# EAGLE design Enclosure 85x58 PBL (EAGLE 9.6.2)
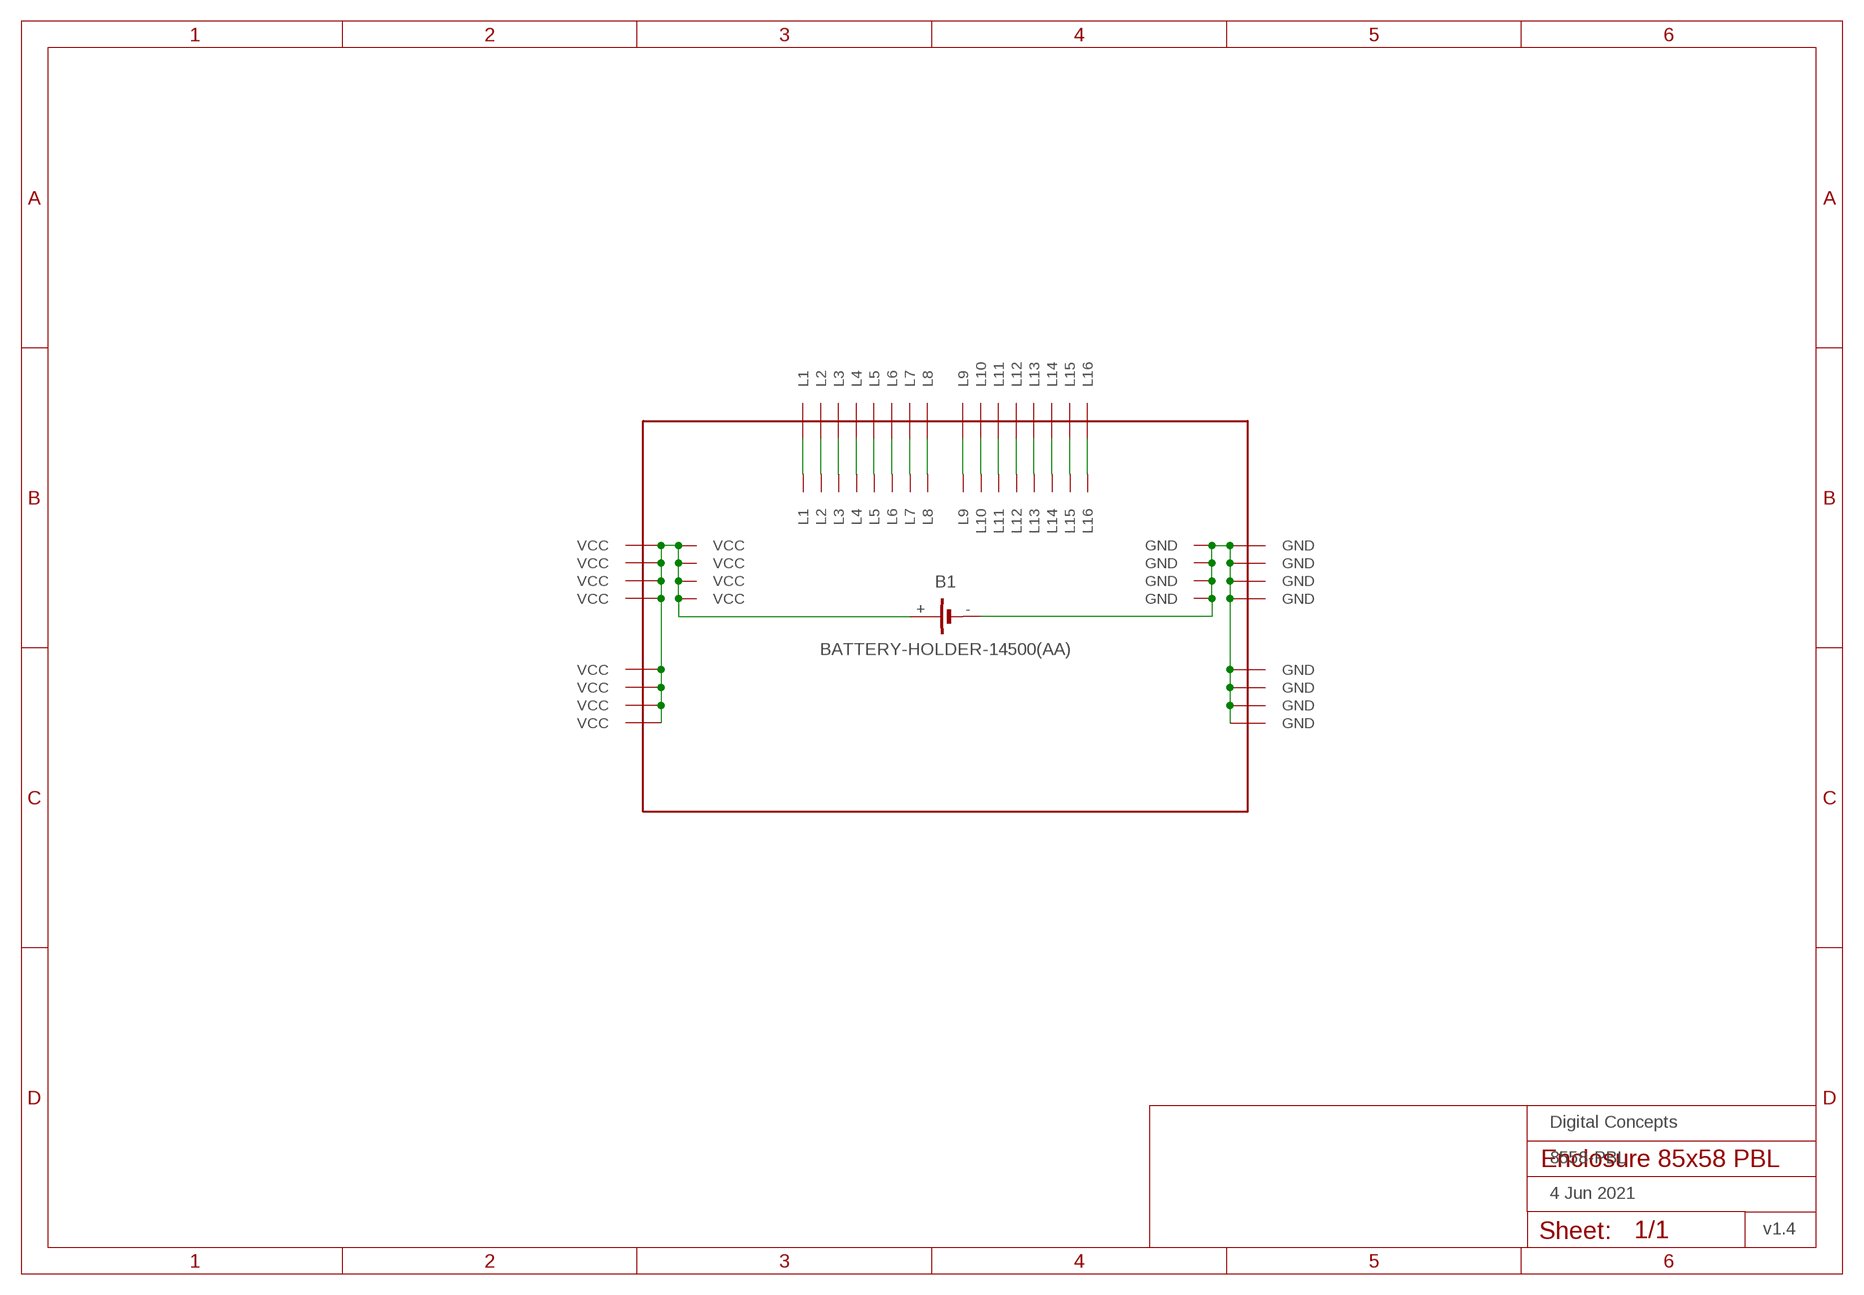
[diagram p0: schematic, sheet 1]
FRAME1 (FRAME-A4L-LOC): DATE: 4 Jun 2021; OWNER: Digital Concepts; TITLE: 8558-PBL; VERSION: v1.4

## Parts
B1  BATTERY-HOLDER-14500(AA)  [BATTERY-14500]
U$1  PROTO-28X18-BAT  [PROTO-28X18-BAT]

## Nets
GND: B1.- U$1.P27-12(GND) U$1.P27-13(GND) U$1.P27-14(GND) U$1.P27-15(GND) U$1.P28-04(GND) U$1.P28-05(GND) U$1.P28-06(GND) U$1.P28-07(GND) U$1.P28-12(GND) U$1.P28-13(GND) U$1.P28-14(GND) U$1.P28-15(GND)
N$4: U$1.P07-17(L1) U$1.P07-18(L1)
N$5: U$1.P08-17(L2) U$1.P08-18(L2)
N$6: U$1.P09-17(L3) U$1.P09-18(L3)
N$7: U$1.P10-17(L4) U$1.P10-18(L4)
N$8: U$1.P11-17(L5) U$1.P11-18(L5)
N$9: U$1.P12-17(L6) U$1.P12-18(L6)
N$10: U$1.P13-17(L7) U$1.P13-18(L7)
N$11: U$1.P14-17(L8) U$1.P14-18(L8)
N$12: U$1.P15-17(L9) U$1.P15-18(L9)
N$13: U$1.P16-17(L10) U$1.P16-18(L10)
N$14: U$1.P17-17(L11) U$1.P17-18(L11)
N$15: U$1.P18-17(L12) U$1.P18-18(L12)
N$16: U$1.P19-17(L13) U$1.P19-18(L13)
N$17: U$1.P20-17(L14) U$1.P20-18(L14)
N$18: U$1.P21-17(L15) U$1.P21-18(L15)
N$19: U$1.P22-17(L16) U$1.P22-18(L16)
VCC: B1.+ U$1.P01-04(VCC) U$1.P01-05(VCC) U$1.P01-06(VCC) U$1.P01-07(VCC) U$1.P01-12(VCC) U$1.P01-13(VCC) U$1.P01-14(VCC) U$1.P01-15(VCC) U$1.P02-12(VCC) U$1.P02-13(VCC) U$1.P02-14(VCC) U$1.P02-15(VCC)

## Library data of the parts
B1 = digitalconcepts:BATTERY-HOLDER-14500(AA): 14500 (AA) battery holder
U$1 = digitalconcepts:PROTO-28X18-BAT: 28 x 18 Prototyping board, with battery connection (GND + Vcc plane) and coupled side connection points, to fit an 85 x 58 enclosure

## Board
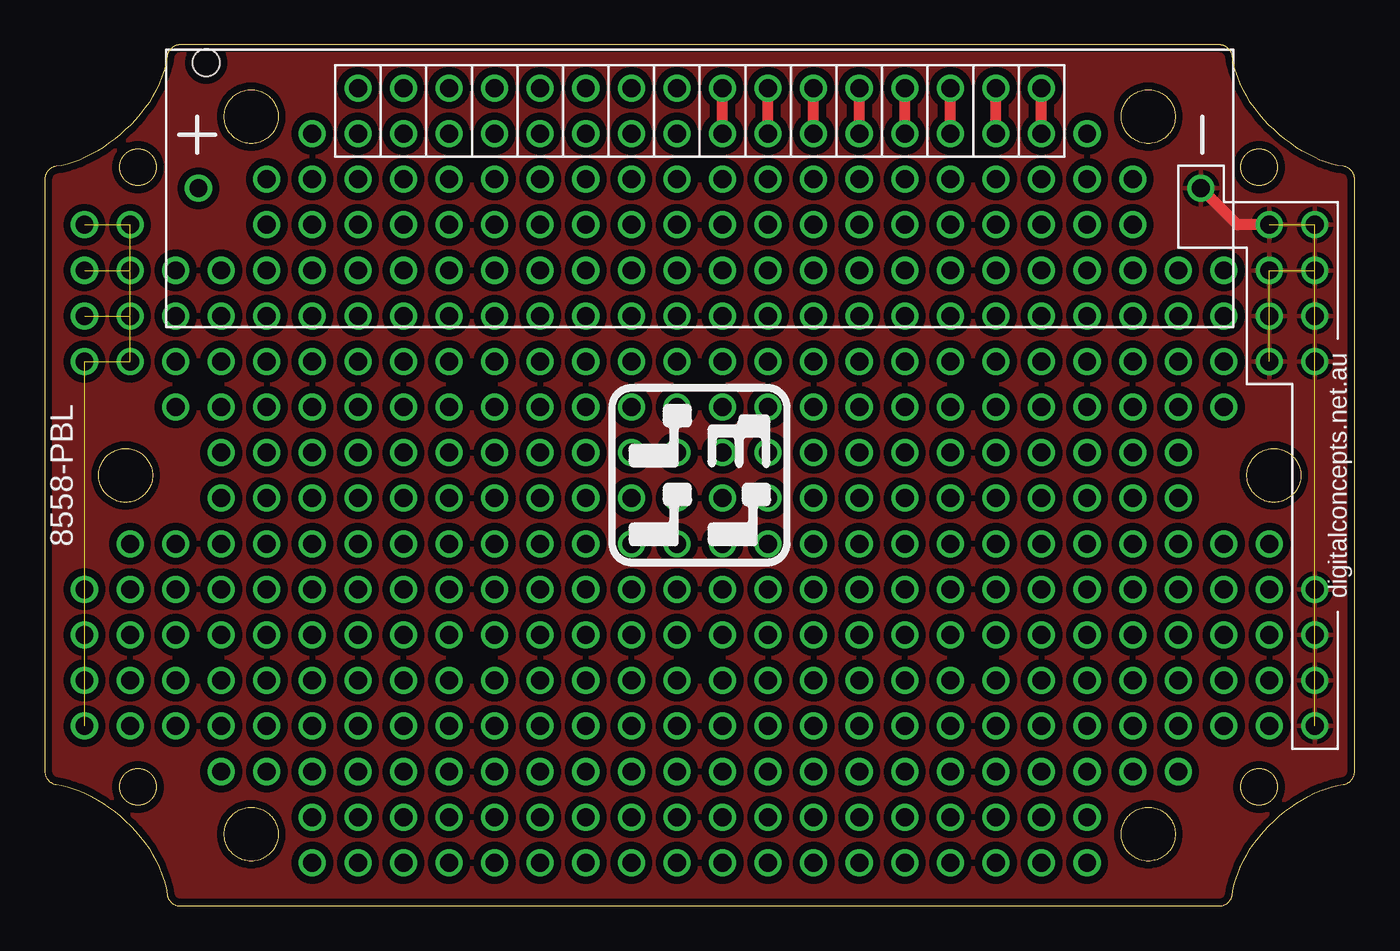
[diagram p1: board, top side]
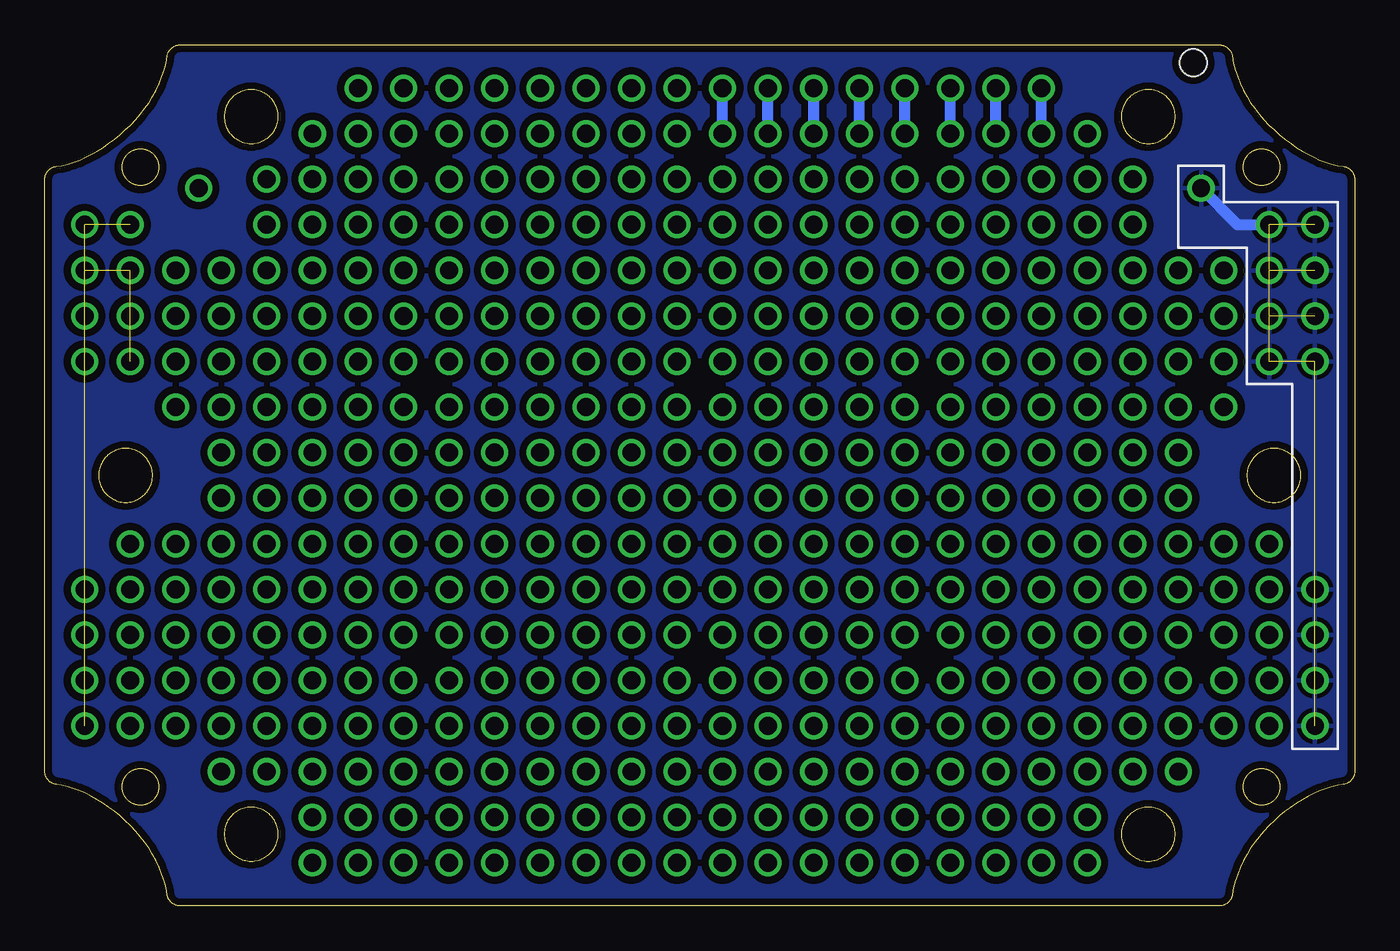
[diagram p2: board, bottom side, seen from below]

Size 73 x 48 mm. Coordinates in mm from the lower left corner, seen from the top.
Outline: 828 segments
Outline: circle at 5.19,41.18 radius 1.02
Outline: circle at 5.19,6.64 radius 1.02
Outline: circle at 67.67,6.64 radius 1.02
Outline: circle at 67.67,41.18 radius 1.02
Copper layers (1*16): Top 0.035mm / dielectric 1.5mm / Bottom 0.035mm
Design rules "default *": minimum track width 6mil, minimum drill 0.35mm, track to track 6mil, track to pad 6mil, pad to pad 6mil, via to via 6mil, smd to smd 6mil, copper to edge 6mil, drill to drill 6mil, minimum pad ring 10mil, minimum via ring 8mil, stop-mask expansion 4mil, vias tented up to drill 0mil, thermal gap 10mil

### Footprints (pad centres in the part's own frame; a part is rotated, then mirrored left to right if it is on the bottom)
BATTERY-14500 = drill 1: + -27.94,0; - 27.94,0 | hole 1.524: -27.5,7
PROTO-28X18-BAT = drill 1: P01-04 -34.29,-13.97; P01-05 -34.29,-11.43; P01-06 -34.29,-8.89; P01-07 -34.29,-6.35; P01-12 -34.29,6.35; P01-13 -34.29,8.89; P01-14 -34.29,11.43; P01-15 -34.29,13.97; P02-04 -31.75,-13.97; P02-05 -31.75,-11.43; P02-06 -31.75,-8.89; P02-07 -31.75,-6.35; P02-08 -31.75,-3.81; P02-12 -31.75,6.35; P02-13 -31.75,8.89; P02-14 -31.75,11.43; P02-15 -31.75,13.97; P03-04 -29.21,-13.97; P03-05 -29.21,-11.43; P03-06 -29.21,-8.89; P03-07 -29.21,-6.35; P03-08 -29.21,-3.81; P03-11 -29.21,3.81; P03-12 -29.21,6.35; P03-13 -29.21,8.89; P03-14 -29.21,11.43; P04-03 -26.67,-16.51; P04-04 -26.67,-13.97; P04-05 -26.67,-11.43; P04-06 -26.67,-8.89; P04-07 -26.67,-6.35; P04-08 -26.67,-3.81; P04-09 -26.67,-1.27; P04-10 -26.67,1.27; P04-11 -26.67,3.81; P04-12 -26.67,6.35; P04-13 -26.67,8.89; P04-14 -26.67,11.43; P05-03 -24.13,-16.51; P05-04 -24.13,-13.97; P05-05 -24.13,-11.43; P05-06 -24.13,-8.89; P05-07 -24.13,-6.35; P05-08 -24.13,-3.81; P05-09 -24.13,-1.27; P05-10 -24.13,1.27; P05-11 -24.13,3.81; P05-12 -24.13,6.35; P05-13 -24.13,8.89; P05-14 -24.13,11.43; P05-15 -24.13,13.97; P05-16 -24.13,16.51; P06-01 -21.59,-21.59; P06-02 -21.59,-19.05; P06-03 -21.59,-16.51; P06-04 -21.59,-13.97; P06-05 -21.59,-11.43; P06-06 -21.59,-8.89; P06-07 -21.59,-6.35; P06-08 -21.59,-3.81; P06-09 -21.59,-1.27; P06-10 -21.59,1.27; P06-11 -21.59,3.81; P06-12 -21.59,6.35; P06-13 -21.59,8.89; P06-14 -21.59,11.43; P06-15 -21.59,13.97; P06-16 -21.59,16.51; P06-17 -21.59,19.05; P07-01 -19.05,-21.59; P07-02 -19.05,-19.05; P07-03 -19.05,-16.51; P07-04 -19.05,-13.97; P07-05 -19.05,-11.43; P07-06 -19.05,-8.89; P07-07 -19.05,-6.35; P07-08 -19.05,-3.81; P07-09 -19.05,-1.27; P07-10 -19.05,1.27; P07-11 -19.05,3.81; P07-12 -19.05,6.35; P07-13 -19.05,8.89; P07-14 -19.05,11.43; P07-15 -19.05,13.97; P07-16 -19.05,16.51; P07-17 -19.05,19.05; P07-18 -19.05,21.59; P08-01 -16.51,-21.59; P08-02 -16.51,-19.05; P08-03 -16.51,-16.51; P08-04 -16.51,-13.97; P08-05 -16.51,-11.43; P08-06 -16.51,-8.89; P08-07 -16.51,-6.35; P08-08 -16.51,-3.81; P08-09 -16.51,-1.27; P08-10 -16.51,1.27; P08-11 -16.51,3.81; P08-12 -16.51,6.35; P08-13 -16.51,8.89; P08-14 -16.51,11.43; P08-15 -16.51,13.97; P08-16 -16.51,16.51; P08-17 -16.51,19.05; P08-18 -16.51,21.59; P09-01 -13.97,-21.59; P09-02 -13.97,-19.05; P09-03 -13.97,-16.51; P09-04 -13.97,-13.97; P09-05 -13.97,-11.43; P09-06 -13.97,-8.89; P09-07 -13.97,-6.35; P09-08 -13.97,-3.81; P09-09 -13.97,-1.27; P09-10 -13.97,1.27; P09-11 -13.97,3.81; P09-12 -13.97,6.35; P09-13 -13.97,8.89; P09-14 -13.97,11.43; P09-15 -13.97,13.97; P09-16 -13.97,16.51; P09-17 -13.97,19.05; P09-18 -13.97,21.59; P10-01 -11.43,-21.59; P10-02 -11.43,-19.05; P10-03 -11.43,-16.51; P10-04 -11.43,-13.97; P10-05 -11.43,-11.43; P10-06 -11.43,-8.89; P10-07 -11.43,-6.35; P10-08 -11.43,-3.81; P10-09 -11.43,-1.27; P10-10 -11.43,1.27; P10-11 -11.43,3.81; P10-12 -11.43,6.35; P10-13 -11.43,8.89; P10-14 -11.43,11.43; P10-15 -11.43,13.97; P10-16 -11.43,16.51; P10-17 -11.43,19.05; P10-18 -11.43,21.59; P11-01 -8.89,-21.59; P11-02 -8.89,-19.05; P11-03 -8.89,-16.51; P11-04 -8.89,-13.97; P11-05 -8.89,-11.43; P11-06 -8.89,-8.89; P11-07 -8.89,-6.35; P11-08 -8.89,-3.81; P11-09 -8.89,-1.27; P11-10 -8.89,1.27; P11-11 -8.89,3.81; P11-12 -8.89,6.35; P11-13 -8.89,8.89; P11-14 -8.89,11.43; P11-15 -8.89,13.97; P11-16 -8.89,16.51; P11-17 -8.89,19.05; P11-18 -8.89,21.59; P12-01 -6.35,-21.59; P12-02 -6.35,-19.05; P12-03 -6.35,-16.51; P12-04 -6.35,-13.97; P12-05 -6.35,-11.43; P12-06 -6.35,-8.89; P12-07 -6.35,-6.35; P12-08 -6.35,-3.81; P12-09 -6.35,-1.27; P12-10 -6.35,1.27; P12-11 -6.35,3.81; P12-12 -6.35,6.35; P12-13 -6.35,8.89; P12-14 -6.35,11.43; P12-15 -6.35,13.97; P12-16 -6.35,16.51; P12-17 -6.35,19.05; P12-18 -6.35,21.59; P13-01 -3.81,-21.59; P13-02 -3.81,-19.05; P13-03 -3.81,-16.51; P13-04 -3.81,-13.97; P13-05 -3.81,-11.43; P13-06 -3.81,-8.89; P13-07 -3.81,-6.35; P13-08 -3.81,-3.81; P13-09 -3.81,-1.27; P13-10 -3.81,1.27; P13-11 -3.81,3.81; P13-12 -3.81,6.35; P13-13 -3.81,8.89; P13-14 -3.81,11.43; P13-15 -3.81,13.97; P13-16 -3.81,16.51; P13-17 -3.81,19.05; P13-18 -3.81,21.59; P14-01 -1.27,-21.59; P14-02 -1.27,-19.05; P14-03 -1.27,-16.51; P14-04 -1.27,-13.97; P14-05 -1.27,-11.43; P14-06 -1.27,-8.89; P14-07 -1.27,-6.35; P14-08 -1.27,-3.81; P14-09 -1.27,-1.27; P14-10 -1.27,1.27; P14-11 -1.27,3.81; P14-12 -1.27,6.35; P14-13 -1.27,8.89; P14-14 -1.27,11.43; P14-15 -1.27,13.97; P14-16 -1.27,16.51; P14-17 -1.27,19.05; P14-18 -1.27,21.59; P15-01 1.27,-21.59; P15-02 1.27,-19.05; P15-03 1.27,-16.51; P15-04 1.27,-13.97; P15-05 1.27,-11.43; P15-06 1.27,-8.89; P15-07 1.27,-6.35; P15-08 1.27,-3.81; P15-09 1.27,-1.27; P15-10 1.27,1.27; P15-11 1.27,3.81; P15-12 1.27,6.35; P15-13 1.27,8.89; P15-14 1.27,11.43; P15-15 1.27,13.97; P15-16 1.27,16.51; P15-17 1.27,19.05; P15-18 1.27,21.59; P16-01 3.81,-21.59; P16-02 3.81,-19.05; P16-03 3.81,-16.51; P16-04 3.81,-13.97; P16-05 3.81,-11.43; P16-06 3.81,-8.89; P16-07 3.81,-6.35; P16-08 3.81,-3.81; P16-09 3.81,-1.27; P16-10 3.81,1.27; P16-11 3.81,3.81; P16-12 3.81,6.35; P16-13 3.81,8.89; P16-14 3.81,11.43; P16-15 3.81,13.97; P16-16 3.81,16.51; P16-17 3.81,19.05; P16-18 3.81,21.59; P17-01 6.35,-21.59; P17-02 6.35,-19.05; P17-03 6.35,-16.51; P17-04 6.35,-13.97; P17-05 6.35,-11.43; P17-06 6.35,-8.89; P17-07 6.35,-6.35; P17-08 6.35,-3.81; P17-09 6.35,-1.27; P17-10 6.35,1.27; P17-11 6.35,3.81; P17-12 6.35,6.35; P17-13 6.35,8.89; P17-14 6.35,11.43; P17-15 6.35,13.97; P17-16 6.35,16.51; P17-17 6.35,19.05; P17-18 6.35,21.59; P18-01 8.89,-21.59; P18-02 8.89,-19.05; P18-03 8.89,-16.51; P18-04 8.89,-13.97; P18-05 8.89,-11.43; P18-06 8.89,-8.89; P18-07 8.89,-6.35; P18-08 8.89,-3.81; P18-09 8.89,-1.27; P18-10 8.89,1.27; P18-11 8.89,3.81; P18-12 8.89,6.35; P18-13 8.89,8.89; P18-14 8.89,11.43; P18-15 8.89,13.97; P18-16 8.89,16.51; P18-17 8.89,19.05; P18-18 8.89,21.59; P19-01 11.43,-21.59; P19-02 11.43,-19.05; P19-03 11.43,-16.51; P19-04 11.43,-13.97; P19-05 11.43,-11.43; P19-06 11.43,-8.89; P19-07 11.43,-6.35; P19-08 11.43,-3.81; P19-09 11.43,-1.27; P19-10 11.43,1.27; P19-11 11.43,3.81; P19-12 11.43,6.35; P19-13 11.43,8.89; P19-14 11.43,11.43; P19-15 11.43,13.97; P19-16 11.43,16.51; P19-17 11.43,19.05; P19-18 11.43,21.59; P20-01 13.97,-21.59; P20-02 13.97,-19.05; P20-03 13.97,-16.51; P20-04 13.97,-13.97; P20-05 13.97,-11.43; P20-06 13.97,-8.89; P20-07 13.97,-6.35; P20-08 13.97,-3.81; P20-09 13.97,-1.27; P20-10 13.97,1.27; P20-11 13.97,3.81; P20-12 13.97,6.35; P20-13 13.97,8.89; P20-14 13.97,11.43; P20-15 13.97,13.97; P20-16 13.97,16.51; P20-17 13.97,19.05; P20-18 13.97,21.59; P21-01 16.51,-21.59; P21-02 16.51,-19.05; P21-03 16.51,-16.51; P21-04 16.51,-13.97; P21-05 16.51,-11.43; P21-06 16.51,-8.89; P21-07 16.51,-6.35; P21-08 16.51,-3.81; P21-09 16.51,-1.27; P21-10 16.51,1.27; P21-11 16.51,3.81; P21-12 16.51,6.35; P21-13 16.51,8.89; P21-14 16.51,11.43; P21-15 16.51,13.97; P21-16 16.51,16.51; P21-17 16.51,19.05; P21-18 16.51,21.59; P22-01 19.05,-21.59; P22-02 19.05,-19.05; P22-03 19.05,-16.51; P22-04 19.05,-13.97; P22-05 19.05,-11.43; P22-06 19.05,-8.89; P22-07 19.05,-6.35; P22-08 19.05,-3.81; P22-09 19.05,-1.27; P22-10 19.05,1.27; P22-11 19.05,3.81; P22-12 19.05,6.35; P22-13 19.05,8.89; P22-14 19.05,11.43; P22-15 19.05,13.97; P22-16 19.05,16.51; P22-17 19.05,19.05; P22-18 19.05,21.59; P23-01 21.59,-21.59; P23-02 21.59,-19.05; P23-03 21.59,-16.51; P23-04 21.59,-13.97; P23-05 21.59,-11.43; P23-06 21.59,-8.89; P23-07 21.59,-6.35; P23-08 21.59,-3.81; P23-09 21.59,-1.27; P23-10 21.59,1.27; P23-11 21.59,3.81; P23-12 21.59,6.35; P23-13 21.59,8.89; P23-14 21.59,11.43; P23-15 21.59,13.97; P23-16 21.59,16.51; P23-17 21.59,19.05; P24-03 24.13,-16.51; P24-04 24.13,-13.97; P24-05 24.13,-11.43; P24-06 24.13,-8.89; P24-07 24.13,-6.35; P24-08 24.13,-3.81; P24-09 24.13,-1.27; P24-10 24.13,1.27; P24-11 24.13,3.81; P24-12 24.13,6.35; P24-13 24.13,8.89; P24-14 24.13,11.43; P24-15 24.13,13.97; P24-16 24.13,16.51; P25-03 26.67,-16.51; P25-04 26.67,-13.97; P25-05 26.67,-11.43; P25-06 26.67,-8.89; P25-07 26.67,-6.35; P25-08 26.67,-3.81; P25-09 26.67,-1.27; P25-10 26.67,1.27; P25-11 26.67,3.81; P25-12 26.67,6.35; P25-13 26.67,8.89; P25-14 26.67,11.43; P26-04 29.21,-13.97; P26-05 29.21,-11.43; P26-06 29.21,-8.89; P26-07 29.21,-6.35; P26-08 29.21,-3.81; P26-11 29.21,3.81; P26-12 29.21,6.35; P26-13 29.21,8.89; P26-14 29.21,11.43; P27-04 31.75,-13.97; P27-05 31.75,-11.43; P27-06 31.75,-8.89; P27-07 31.75,-6.35; P27-08 31.75,-3.81; P27-12 31.75,6.35; P27-13 31.75,8.89; P27-14 31.75,11.43; P27-15 31.75,13.97; P28-04 34.29,-13.97; P28-05 34.29,-11.43; P28-06 34.29,-8.89; P28-07 34.29,-6.35; P28-12 34.29,6.35; P28-13 34.29,8.89; P28-14 34.29,11.43; P28-15 34.29,13.97

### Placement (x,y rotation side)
B1  36.5,40 0 top
U$1  36.5,24 0 top

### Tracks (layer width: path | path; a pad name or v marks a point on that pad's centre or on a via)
GND  (11 unrouted)
  Top 0.61: U$1.P27-15 66.47,37.97 B1.-
  pour Top (isolate 0.406): -1.6,50.03 75.11,50.03 75.11,-1.78 -1.6,-1.78
N$4
  Bottom 0.6: U$1.P07-17 U$1.P07-18
N$5
  Bottom 0.6: U$1.P08-17 U$1.P08-18
N$6
  Bottom 0.6: U$1.P09-17 U$1.P09-18
N$7
  Bottom 0.6: U$1.P10-17 U$1.P10-18
N$8
  Bottom 0.6: U$1.P11-17 U$1.P11-18
N$9
  Bottom 0.6: U$1.P12-17 U$1.P12-18
N$10
  Bottom 0.6: U$1.P13-17 U$1.P13-18
N$11
  Bottom 0.6: U$1.P14-17 U$1.P14-18
N$12
  Top 0.6: U$1.P15-17 U$1.P15-18
N$13
  Top 0.6: U$1.P16-17 U$1.P16-18
N$14
  Top 0.6: U$1.P17-17 U$1.P17-18
N$15
  Top 0.6: U$1.P18-17 U$1.P18-18
N$16
  Top 0.6: U$1.P19-17 U$1.P19-18
N$17
  Top 0.6: U$1.P20-17 U$1.P20-18
N$18
  Top 0.6: U$1.P21-17 U$1.P21-18
N$19
  Top 0.6: U$1.P22-17 U$1.P22-18
VCC  (11 unrouted)
  Bottom 0.61: B1.+ 6.53,37.97 U$1.P02-15
  pour Bottom (isolate 0.406): -0.33,48.76 73.84,48.76 73.84,-0.51 -0.33,-0.51

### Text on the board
tPlace: 8558-PBL | digitalconcepts.net.au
